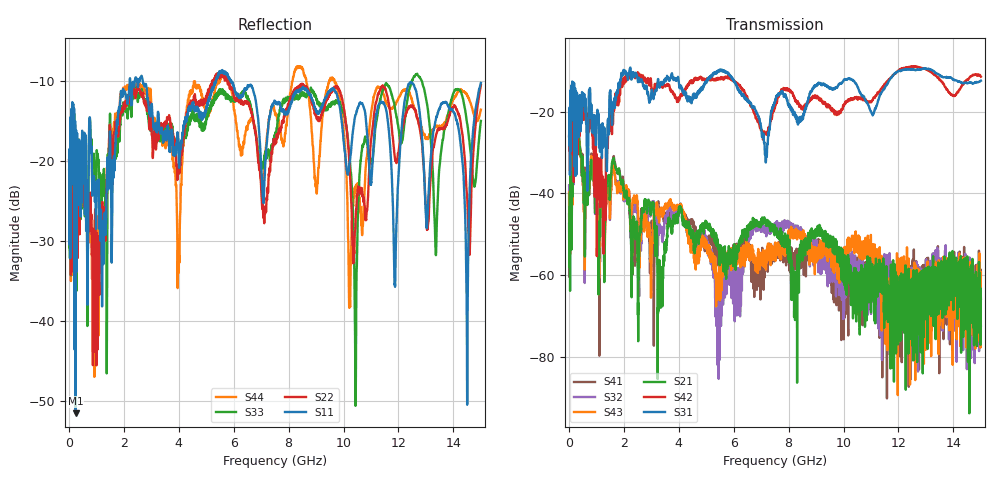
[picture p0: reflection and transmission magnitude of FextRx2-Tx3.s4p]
! FILE: N:\QM 2007\Prüfprotokolle\Highspeed\Konfektionierte Ltg\L45593-D106\D30\8216\0002\Fext\FextRx2-Tx3.s4p
# MHz S DB R 50.00
! FREQ  S11  S12  S13  S14
!  S21  S22  S23  S24
!  S31  S32  S33  S34
!  S41  S42  S43  S44
!  DB  ANG  DB  ANG  DB  ANG  DB  ANG
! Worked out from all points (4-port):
!   2999 points, 10 MHz to 15 GHz, reference 50 ohm
!   strongest paths, dB at 10 MHz, 3.755 GHz, 7.505 GHz, 11.26 GHz, 15 GHz:
!     S31: -25.8, -10.5, -17.3, -17.3, -12.4
!     S42: -26.1, -15.1, -18.9, -15.6, -11.4
!     S21: -47.5, -48.7, -49.2, -59.6, -65.8
!     S43: -39.9, -43.4, -55.5, -55.3, -59.4
!     S32: -38.0, -45.6, -48.1, -62.4, -72.4
!     S41: -45.1, -45.6, -52.3, -57.8, -59.9
!   lowest |S11| = -51.6 dB at 245 MHz (marker M1), VSWR 1.01, Z = 50.1 + j0.249 ohm
!   |S11| at or under -10 dB: start of sweep to 2.215 GHz; 2.692 GHz to 5.334 GHz (2.642 GHz wide, 65.8 % of centre); 5.924 GHz to end of sweep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
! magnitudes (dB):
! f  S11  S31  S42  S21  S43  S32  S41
! 10 MHz  -19.8  -25.8  -26.1  -47.5  -39.9  -38.0  -45.1
! 245 MHz  -51.6  -35.7  -21.0  -27.9  -28.3  -28.2  -27.2
! 5.45 GHz  -9.0  -10.2  -12.1  -53.7  -62.6  -65.0  -55.9
! 9.86 GHz  -13.2  -13.1  -20.3  -55.5  -56.5  -57.3  -56.0
! 10.43 GHz  -14.2  -13.0  -16.4  -67.7  -49.5  -58.8  -59.7
! 14.49 GHz  -47.7  -12.9  -12.2  -69.0  -57.7  -59.6  -59.0
! 15 GHz  -10.2  -12.4  -11.4  -65.8  -59.4  -72.4  -59.9
